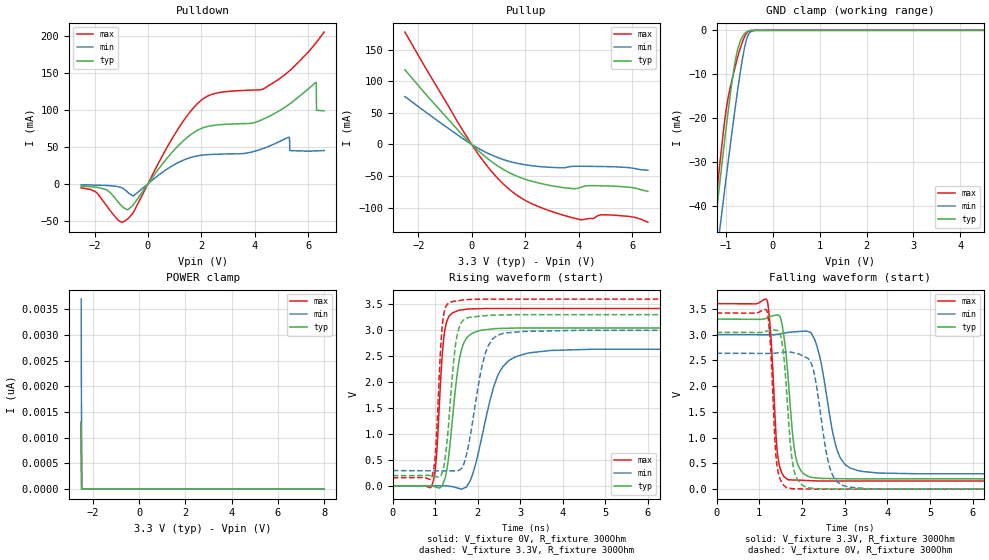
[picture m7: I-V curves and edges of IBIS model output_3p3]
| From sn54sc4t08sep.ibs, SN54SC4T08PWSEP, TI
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|   output_3p3 Model
[Model]   output_3p3
Model_type   3-state
Polarity   Non-Inverting
Vmeas = 1.65
Vref = 0
Cref = 2pF
Rref = 100000
|   typ   min   max
C_comp   5.7pF   5.6pF   6pF
[Voltage Range]   3.3   3   3.6
[Temperature Range]   25   125   -40
[Pullup Reference]   3.3   3   3.6
[Pulldown Reference]   0   0   0
[Power Clamp Reference]   3.3   3   3.6
[GND Clamp Reference]   0   0   0
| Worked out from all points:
|   slope of the pulldown table from 0 to 0.495 V, typ, clamps not added: 20 ohm
|   slope of the pullup table from 0 to 0.495 V, typ, clamps not added: 26.3 ohm
|   GND clamp passes 1 mA (typ) near -0.62 V on its own axis
|   falling waveform, V_fixture 3.3V, R_fixture 300Ohm: 20-80 % time 197ps typ, 351ps min, 132ps max; typ from 3.3 V to 0.199 V
|   rising waveform, V_fixture 0V, R_fixture 300Ohm: 20-80 % time 245ps typ, 481ps min, 148ps max; typ from 0 V to 3.04 V
|   rising waveform, V_fixture 3.3V, R_fixture 300Ohm: 20-80 % time 197ps typ, 351ps min, 127ps max; typ from 0.199 V to 3.3 V
|   falling waveform, V_fixture 0V, R_fixture 300Ohm: 20-80 % time 173ps typ, 299ps min, 121ps max; typ from 3.04 V to 0 V
[Pulldown]
|   Voltage   I(typ)   I(min)   I(max)
-2.5V     -3.063mA   -1.274mA   -5.409mA
-1.555V   -7.805mA   -2.184mA   -29.26mA
-914.5mV  -32.18mA   -6.478mA   -51.06mA
-547mV    -28.32mA   -16.32mA   -38.72mA
1.899V    73.17mA    38.13mA    110mA
4.293V    87.03mA    47.49mA    127.7mA
5.27V     107mA      63.02mA    151.7mA
5.312V    108.1mA    45.03mA    153mA
6.288V    137mA      44.47mA    190.3mA
6.299V    136.5mA    44.48mA    190.8mA
6.309V    99.3mA     44.5mA     191.3mA
6.593V    98.6mA     45.03mA    204.9mA
[GND Clamp]
|   Voltage   I(typ)   I(min)   I(max)
-2.5V     -170.7mA   -168.9mA   -187.4mA
-1.282V   -49.09mA   -58.54mA   -46.61mA
-1.24V    -45.04mA   -54.83mA   -42.02mA
-1.208V   -42.02mA   -52.06mA   -38.61mA
-1.125V   -34.05mA   -44.71mA   -29.82mA
-977.5mV  -20.62mA   -32.07mA   -16.86mA
-799mV    -6.847mA   -17.4mA    -8.124mA
-715mV    -3.091mA   -11.05mA   -4.817mA
-641.5mV  -1.357mA   -6.134mA   -2.454mA
-526mV    -161.3uA   -1.092mA   -287.1uA
-379mV    -1.458uA   -24.15uA   -787.7nA
8V        0A         0A         0A
[Pullup]
|   Voltage   I(typ)   I(min)   I(max)
-2.5V     118mA      75.5mA     177.6mA
-547mV    24.12mA    15.55mA    36.89mA
135.5mV   -5.49mA    -3.436mA   -8.61mA
870.5mV   -30.97mA   -18.98mA   -48.86mA
1.574V    -48.08mA   -28.66mA   -76.64mA
2.487V    -60.77mA   -34.76mA   -98.07mA
3.958V    -69.51mA   -34.5mA    -117.8mA
4.252V    -65.52mA   -34.58mA   -118.2mA
4.819V    -65.37mA   -34.9mA    -111.4mA
5.133V    -65.75mA   -35.13mA   -111.4mA
6.026V    -68.37mA   -37.5mA    -114.7mA
6.593V    -74.29mA   -40.79mA   -122.9mA
[POWER Clamp]
|   Voltage   I(typ)   I(min)   I(max)
-2.5V     1.265nA    3.699nA    1.306nA
-2.479V   0A         0A         0A
-2.469V   0A         0A         0A
8V        0A         0A         0A
[Ramp]
R_load = 300
|   typ   min   max
dV/dt_r   1.82626/2.43663e-10   1.58192/4.79856e-10   2.05136/1.48099e-10
dV/dt_f   1.86048/1.96516e-10   1.62221/3.4876e-10   2.06543/1.32346e-10
[Falling Waveform]
V_fixture = 3.3V
V_fixture_min = 3V
V_fixture_max = 3.6V
R_fixture = 300Ohm
C_fixture = 0F
|   Time   V(typ)   V(min)   V(max)
0s        3.3V       3V         3.6V
1.179ns   3.322V     2.996V     3.67V
1.43ns    3.38V      3.007V     657.9mV
1.668ns   2.232V     3.04V      186.2mV
1.82ns    788.5mV    3.053V     177.8mV
1.983ns   349.6mV    3.062V     172.3mV
2.353ns   217mV      2.764V     160mV
2.851ns   203.9mV    692.2mV    157.9mV
3.311ns   199.9mV    359.5mV    157.9mV
15ns      199.2mV    296.3mV    157.6mV
[Rising Waveform]
V_fixture = 0V
V_fixture_min = 0V
V_fixture_max = 0V
R_fixture = 300Ohm
C_fixture = 0F
|   Time   V(typ)   V(min)   V(max)
0s        3.096uV    497.8nV    4.463uV
928.6ps   -1.847mV   1.398mV    25.11mV
1.022ns   -24.45mV   1.539mV    519.4mV
1.153ns   -360.9uV   1.736mV    2.399V
1.22ns    124.7mV    1.837mV    2.979V
1.541ns   2.31V      -44.37mV   3.379V
1.872ns   2.942V     210.2mV    3.412V
2.489ns   3.033V     2.159V     3.418V
3.143ns   3.042V     2.552V     3.418V
15ns      3.044V     2.637V     3.419V
[Rising Waveform]
V_fixture = 3.3V
V_fixture_min = 3V
V_fixture_max = 3.6V
R_fixture = 300Ohm
C_fixture = 0F
|   Time   V(typ)   V(min)   V(max)
0s        199.2mV    296.3mV    157.6mV
922.9ps   198.9mV    291.4mV    182.5mV
1.01ns    181.6mV    290.9mV    729.9mV
1.174ns   281.8mV    290.1mV    3.155V
1.39ns    2.012V     288.9mV    3.549V
1.5ns     2.841V     289.9mV    3.564V
1.628ns   3.167V     349.1mV    3.58V
2.171ns   3.279V     2.538V     3.599V
2.593ns   3.294V     2.938V     3.599V
15ns      3.3V       3V         3.6V
[Falling Waveform]
|Gnd
V_fixture = 0V
V_fixture_min = 0V
V_fixture_max = 0V
R_fixture = 300Ohm
C_fixture = 0F
|   Time   V(typ)   V(min)   V(max)
0s        3.044V     2.637V     3.419V
1.179ns   3.068V     2.634V     3.46V
1.404ns   3.082V     2.643V     527.2mV
1.646ns   1.825V     2.662V     26.79mV
1.757ns   643mV      2.656V     11.95mV
1.912ns   159.5mV    2.626V     5.908mV
2.252ns   16.67mV    2.356V     1.708mV
2.67ns    4.073mV    367.2mV    389.4uV
3.076ns   842.5uV    43.19mV    376.7uV
15ns      3.363uV    998.2nV    4.521uV
